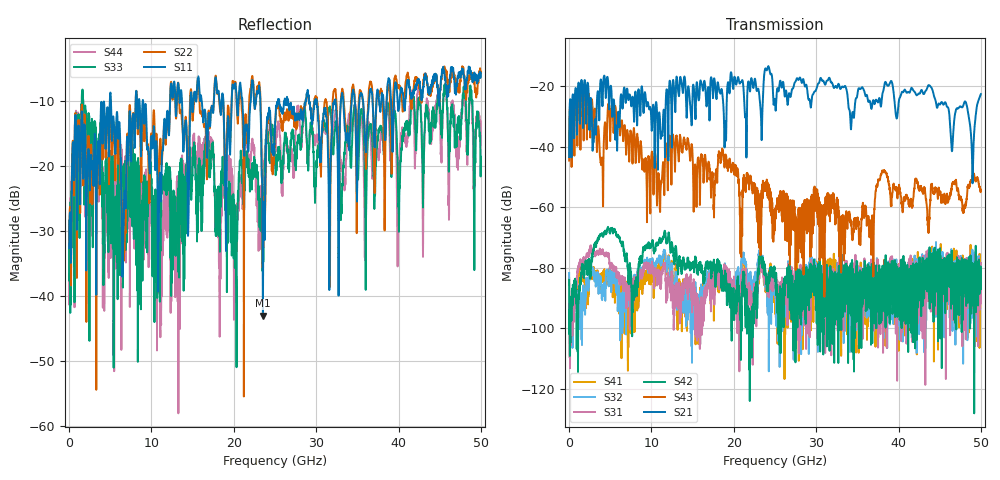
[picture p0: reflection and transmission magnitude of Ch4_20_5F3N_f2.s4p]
!Agilent Technologies,N5247A,US51170199,A.09.90.13
!Agilent N5247A: A.09.90.13
!Date: Monday, December 14, 2015 15:38:08
!Correction: S11(Full 4 Port(1,2,3,4))
!S12(Full 4 Port(1,2,3,4))
!S13(Full 4 Port(1,2,3,4))
!S14(Full 4 Port(1,2,3,4))
!S21(Full 4 Port(1,2,3,4))
!S22(Full 4 Port(1,2,3,4))
!S23(Full 4 Port(1,2,3,4))
!S24(Full 4 Port(1,2,3,4))
!S31(Full 4 Port(1,2,3,4))
!S32(Full 4 Port(1,2,3,4))
!S33(Full 4 Port(1,2,3,4))
!S34(Full 4 Port(1,2,3,4))
!S41(Full 4 Port(1,2,3,4))
!S42(Full 4 Port(1,2,3,4))
!S43(Full 4 Port(1,2,3,4))
!S44(Full 4 Port(1,2,3,4))
!S4P File: Measurements: <S11,S12,S13,S14>,
!<S21,S22,S23,S24>,
!<S31,S32,S33,S34>,
!<S41,S42,S43,S44>:
# Hz S  dB  R 50
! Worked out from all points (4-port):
!   3201 points, 10 MHz to 50 GHz, reference 50 ohm
!   strongest paths, dB at 10 MHz, 12.51 GHz, 25 GHz, 37.5 GHz, 50 GHz:
!     S21: -43.4, -28.3, -25.6, -25.4, -22.6
!     S43: -44.6, -39.3, -62.9, -51.9, -54.6
!     S42: -84.0, -71.8, -83.6, -84.5, -86.9
!     S31: -92.0, -85.6, -83.0, -92.0, -78.5
!     S32: -81.8, -80.5, -90.0, -81.9, -84.3
!     S41: -83.3, -79.0, -84.4, -88.5, -78.5
!   lowest |S11| = -43.0 dB at 23.54 GHz (marker M1), VSWR 1.01, Z = 49.4 - j0.313 ohm
!   |S11| at or under -10 dB: start of sweep to 4.951 GHz; 5.089 GHz to 8.084 GHz (2.995 GHz wide, 45.5 % of centre); 8.994 GHz to 12.27 GHz (3.272 GHz wide, 30.8 % of centre)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
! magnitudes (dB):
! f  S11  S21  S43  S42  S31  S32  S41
! 10 MHz  -32.6  -43.4  -44.6  -84.0  -92.0  -81.8  -83.3
! 12.59 GHz  -9.5  -19.0  -36.0  -74.4  -90.3  -87.7  -82.6
! 22.97 GHz  -8.5  -20.9  -59.1  -81.5  -81.1  -77.5  -83.9
! 23.54 GHz  -43.0  -24.1  -51.3  -78.4  -80.5  -78.8  -80.6
! 43.77 GHz  -8.4  -19.8  -61.7  -73.3  -86.6  -78.8  -78.3
! 48.97 GHz  -6.9  -49.3  -49.8  -82.3  -88.9  -74.1  -79.0
! 50 GHz  -5.7  -22.6  -54.6  -86.9  -78.5  -84.3  -78.5
